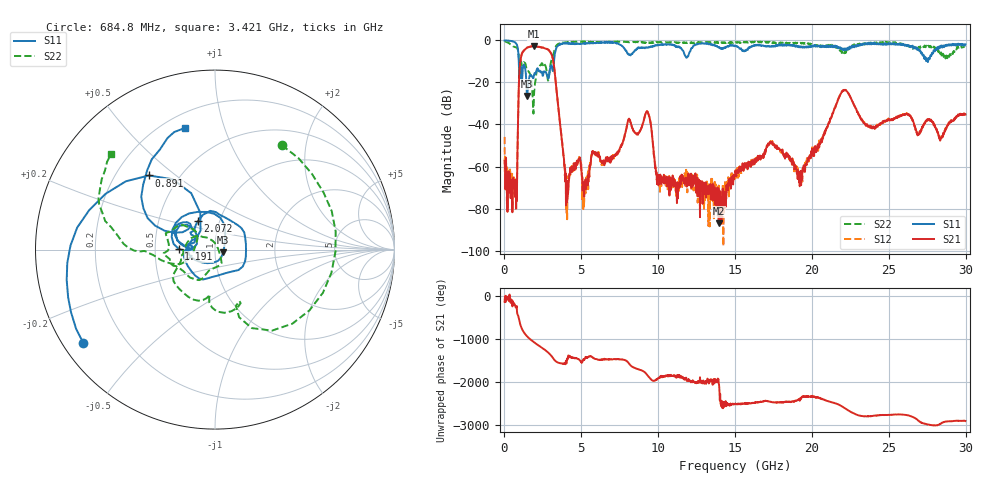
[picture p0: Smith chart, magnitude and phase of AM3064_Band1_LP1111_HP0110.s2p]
# Hz S DB R 50.0
!freq dBS11 angS11 dBS21 angS21 dBS12 angS12 dBS22 angS22
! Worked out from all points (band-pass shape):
!   1600 points, 10 MHz to 29.98 GHz, reference 50 ohm
!   highest |S21| = -2.77 dB at 1.903 GHz (marker M1); lowest = -87.0 dB at 13.94 GHz (marker M2)
!   |S21| within 3 dB of the highest: 1.171 GHz to 2.998 GHz (1.827 GHz wide, 87.6 % of centre)
!   lowest |S11| = -26.4 dB at 1.472 GHz (marker M3), VSWR 1.10, Z = 54.8 - j1.57 ohm
!   |S11| at or under -10 dB: 931.7 MHz to 3.221 GHz (2.289 GHz wide, 110 % of centre); 27.52382 GHz to 27.55056 GHz (26.74 MHz wide, 0.0971 % of centre)
!   |S22| runs from -34.8 to -0.2 dB; largest |S21 - S12| = 0.012
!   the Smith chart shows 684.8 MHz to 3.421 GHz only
!   S11 on the Smith chart (normalised r, x): 684.8 MHz: 0.06, -0.32; 891 MHz: 0.34, +0.40; 1.191 GHz: 0.66, +0.01; 2.072 GHz: 0.79, +0.26; 3.421 GHz: 0.28, +0.75
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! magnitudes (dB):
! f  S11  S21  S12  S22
! 10 MHz  -0.1  -57.3  -45.9  -0.2
! 684.8 MHz  -0.9  -74.5  -70.2  -3.2
! 891 MHz  -5.1  -35.5  -35.3  -5.2
! 1.191 GHz  -13.9  -5.5  -5.5  -11.2
! 1.472 GHz  -26.4  -3.4  -3.4  -14.1
! 1.903 GHz  -17.2  -2.8  -2.8  -30.2
! 2.072 GHz  -14.7  -2.9  -2.9  -15.7
! 3.028 GHz  -12.0  -6.2  -6.1  -10.2
! 3.421 GHz  -3.1  -26.4  -26.3  -2.1
! 4.04 GHz  -1.5  -72.7  -82.1  -0.9
! 5.015 GHz  -1.5  -63.5  -63.5  -0.6
! 9.269 GHz  -3.3  -33.8  -33.6  -1.2
! 10 GHz  -2.2  -68.8  -68.3  -0.9
! 13.94 GHz  -3.2  -87.0  -69.1  -1.0
! 15 GHz  -2.6  -64.6  -65.8  -1.2
! 17.27 GHz  -3.1  -48.3  -48.3  -1.1
! 19.26 GHz  -3.2  -62.1  -66.9  -1.2
! 19.99 GHz  -3.1  -53.6  -53.5  -1.7
! 22.07 GHz  -4.0  -23.7  -23.5  -6.6
! 25 GHz  -1.3  -37.8  -37.7  -1.1
! 28.39 GHz  -2.7  -46.6  -46.5  -5.7
! 29.98 GHz  -1.9  -35.3  -35.3  -2.9
